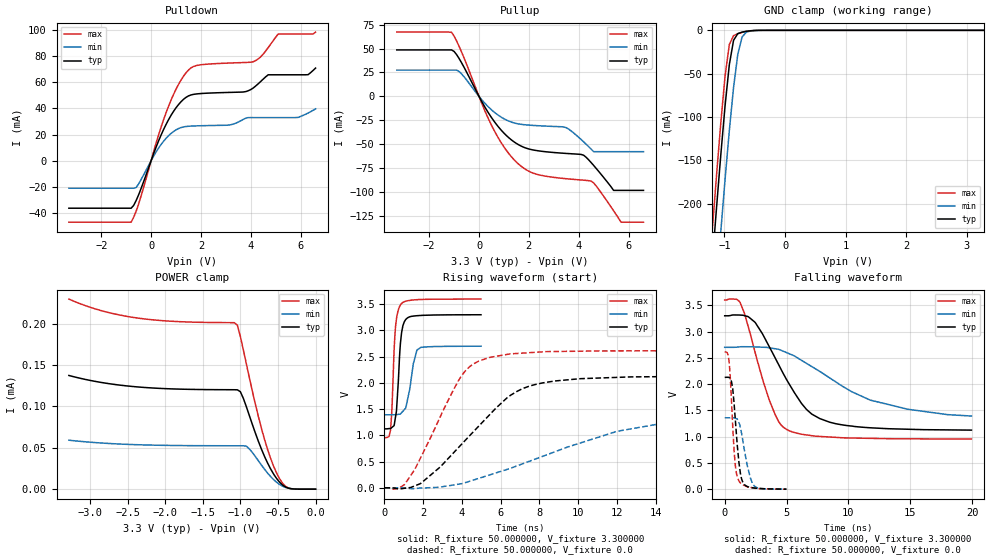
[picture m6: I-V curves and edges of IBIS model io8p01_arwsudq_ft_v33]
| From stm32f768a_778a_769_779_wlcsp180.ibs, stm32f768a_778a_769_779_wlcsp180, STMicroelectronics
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|   Model io8p01_arwsudq_ft_v33
[Model]  io8p01_arwsudq_ft_v33
Model_type I/O
Polarity   Non-Inverting
Enable   Active-Low
Vinl =   0.990000V
Vinh =   2.310000V
Vmeas =  1.650000V
Cref =   50.000000pF
Rref =   100.000000M
Vref =   0.0V
C_comp   2.911600pF   2.826700pF   2.983100pF
[Temperature Range]   25.000000   0.125000k   -40.000000
[Pullup Reference]   3.300000V   2.700000V   3.600000V
[Pulldown Reference]   0.0V   0.0V   0.0V
[POWER Clamp Reference]   3.300000V   2.700000V   3.600000V
[GND Clamp Reference]   0.0V   0.0V   0.0V
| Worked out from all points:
|   slope of the pulldown table from 0 to 0.495 V, typ, clamps not added: 20.9 ohm
|   slope of the pullup table from 0 to 0.495 V, typ, clamps not added: 22.6 ohm
|   GND clamp passes 1 mA (typ) near -0.62 V on its own axis
|   rising waveform, R_fixture 50.000000, V_fixture 3.300000: 20-80 % time 220ps typ, 367ps min, 189ps max; typ from 1.12 V to 3.3 V
|   rising waveform, R_fixture 50.000000, V_fixture 0.0: 20-80 % time 3.34ns typ, 6.51ns min, 2.1ns max; typ from 0 V to 2.13 V
|   falling waveform, R_fixture 50.000000, V_fixture 3.300000: 20-80 % time 3.2ns typ, 6.18ns min, 2.04ns max; typ from 3.3 V to 1.12 V
|   falling waveform, R_fixture 50.000000, V_fixture 0.0: 20-80 % time 464ps typ, 672ps min, 373ps max; typ from 2.13 V to 0 V
[Pulldown]
|Voltage   I(typ)   I(min)   I(max)
-3.3V     -36.38mA   -21.07mA   -47.08mA
-800mV    -36.38mA   -21.07mA   -47.08mA
-600mV    -30.5mA    -20.54mA   -38.69mA
700mV     31.4mA     19.11mA    41.71mA
1.2V      45.15mA    25.37mA    61.75mA
1.6V      50.35mA    26.5mA     71.06mA
3.1V      52.28mA    27.26mA    74.76mA
4.1V      55.71mA    33.02mA    75.8mA
4.7V      65.8mA     33.02mA    86.64mA
5.1V      65.8mA     33.02mA    97.03mA
6.3V      65.87mA    36.5mA     97.03mA
6.6V      70.93mA    39.72mA    98.49mA
[Pullup]
|Voltage   I(typ)   I(min)   I(max)
-3.3V     48.52mA    27.43mA    67.14mA
-1.1V     48.52mA    27.43mA    66.86mA
-700mV    35.13mA    23.48mA    46.33mA
500mV     -22.07mA   -14mA      -30.03mA
1.5V      -49.1mA    -28.3mA    -68.56mA
2.2V      -56.05mA   -30.32mA   -80.35mA
3.5V      -59.53mA   -32.66mA   -85.92mA
4.2V      -61.45mA   -47.47mA   -87.46mA
4.5V      -69.1mA    -55.02mA   -88.4mA
5.4V      -98.1mA    -57.7mA    -119.3mA
5.7V      -98.1mA    -57.7mA    -131.3mA
6.6V      -98.1mA    -57.7mA    -131.3mA
[GND_clamp]
|Voltage   I(typ)   I(min)   I(max)
-3.3V     -2.32A     -2.397A    -2.297A
-1.2V     -266.4mA   -356.3mA   -229.4mA
-1.13V    -203.6mA   -293.1mA   -166.3mA
-1.06V    -143.2mA   -231.4mA   -106.2mA
-990mV    -86.95mA   -171.8mA   -52.65mA
-920mV    -39.66mA   -115.8mA   -16.36mA
-850mV    -11.49mA   -65.84mA   -6.11mA
-780mV    -3.834mA   -27.59mA   -3.88mA
-710mV    -2.09mA    -7.753mA   -2.381mA
-640mV    -1.147mA   -2.129mA   -1.22mA
-570mV    -523.9uA   -800uA     -476.8uA
3.28V     0A         0A         0A
[POWER_clamp]
|Voltage   I(typ)   I(min)   I(max)
-3.28V    137.3uA    59.14uA    229.6uA
-2.36V    123.4uA    53.65uA    206.6uA
-1.08V    120.1uA    52.41uA    201.1uA
-1.04V    120uA      52.41uA    198uA
-1V       117.7uA    52.4uA     184.5uA
-920mV    99.46uA    51.91uA    151.2uA
-720mV    48.42uA    29.12uA    73.51uA
-600mV    24.82uA    15.47uA    37.72uA
-520mV    13.1uA     8.45uA     19.84uA
-440mV    5.058uA    3.61uA     7.276uA
-360mV    1.193uA    1.129uA    1.311uA
0V        0A         0A         0A
[Ramp]
| variable   typ   min   max
dV/dt_r  1.27764/3.33745n   0.80118/6.61556n   1.56792/2.10003n
dV/dt_f  1.30266/3.20888n   0.74232/6.18626n   1.58789/2.03609n
R_load = 50.000000
[Rising Waveform]
R_fixture= 50.000000
V_fixture= 3.300000
V_fixture_min= 2.700000
V_fixture_max= 3.600000
|time   V(typ)   V(min)   V(max)
0s        1.124V     1.392V     954.2mV
320.3ps   1.132V     1.392V     1.122V
390.4ps   1.153V     1.391V     1.53V
500.5ps   1.187V     1.391V     2.641V
620.6ps   1.466V     1.396V     3.219V
850.9ps   2.845V     1.418V     3.499V
1.101ns   3.21V      1.522V     3.558V
1.491ns   3.274V     2.366V     3.582V
1.682ns   3.282V     2.626V     3.587V
4.985ns   3.3V       2.7V       3.599V
[Rising Waveform]
R_fixture= 50.000000
V_fixture= 0.0
V_fixture_min= 0.0
V_fixture_max= 0.0
|time   V(typ)   V(min)   V(max)
0s        198.9uV    84.42uV    722.9uV
1.041ns   -9.237mV   -4.564mV   62.38mV
1.882ns   85.08mV    -4.088mV   582.9mV
3.804ns   759.5mV    67.3mV     2.033V
4.885ns   1.182V     181mV      2.418V
6.527ns   1.768V     374.1mV    2.554V
8.168ns   2V         599.7mV    2.593V
12.01ns   2.105V     1.077V     2.611V
14.77ns   2.12V      1.256V     2.611V
19.94ns   2.129V     1.359V     2.612V
[Falling Waveform]
R_fixture= 50.000000
V_fixture= 3.300000
V_fixture_min= 2.700000
V_fixture_max= 3.600000
|time   V(typ)   V(min)   V(max)
0s        3.3V       2.7V       3.599V
1.241ns   3.313V     2.709V     3.553V
2.442ns   3.178V     2.707V     2.617V
3.604ns   2.711V     2.691V     1.695V
4.364ns   2.368V     2.661V     1.284V
5.045ns   2.067V     2.595V     1.131V
6.607ns   1.519V     2.395V     1.032V
8.488ns   1.274V     2.117V     992.6mV
11.77ns   1.168V     1.694V     967.1mV
19.94ns   1.124V     1.392V     954.2mV
[Falling Waveform]
R_fixture= 50.000000
V_fixture= 0.0
V_fixture_min= 0.0
V_fixture_max= 0.0
|time   V(typ)   V(min)   V(max)
0s        2.129V     1.359V     2.612V
340.3ps   2.125V     1.358V     2.462V
550.6ps   2.047V     1.358V     1.678V
680.7ps   1.833V     1.358V     1.045V
840.8ps   1.376V     1.35V      495.4mV
1.101ns   627.6mV    1.29V      181.8mV
1.461ns   137mV      930.2mV    85.1mV
1.832ns   50.14mV    443mV      45.72mV
2.362ns   23.49mV    68.78mV    20.21mV
4.985ns   198.9uV    84.42uV    722.9uV
